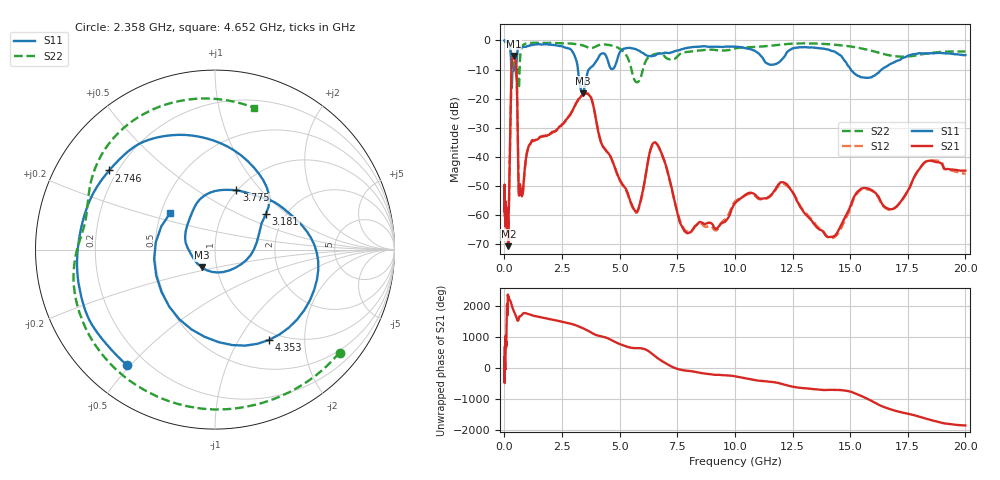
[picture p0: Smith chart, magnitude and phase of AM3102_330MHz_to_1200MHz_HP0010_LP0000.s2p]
! Date/Time: Tue, Sep 11, 2018 5:10 PM
! Network Analyzer: Agilent Technologies E8362B Rev: A.07.50.63
! Sweep from 0.010 to 20.000 GHz, 1601 Points, Sweep Type: LOG
! Power Supply: 4.949 V, 0.000 A
# Hz S DB R 50
!freq MagS11 AngS11 MagS21 AngS21 MagS12 AngS12 MagS22 AngS22
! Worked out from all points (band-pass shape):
!   1601 points, 10 MHz to 20 GHz, reference 50 ohm
!   highest |S21| = -5.33 dB at 402.8 MHz (marker M1); lowest = -70.8 dB at 172.9 MHz (marker M2)
!   |S21| within 3 dB of the highest: 318.5 MHz to 511.9 MHz (193.4 MHz wide, 46.6 % of centre)
!   lowest |S11| = -18.1 dB at 3.4 GHz (marker M3), VSWR 1.28, Z = 42.3 - j8.53 ohm
!   |S11| at or under -10 dB: 298 MHz to 356.1 MHz (58.13 MHz wide, 17.8 % of centre); 3.19 GHz to 3.661 GHz (470.9 MHz wide, 13.7 % of centre); 15.03 GHz to 16.37 GHz (1.347 GHz wide, 8.58 % of centre)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
!   |S22| runs from -16.6 to -0.2 dB; largest |S21 - S12| = 0.0066
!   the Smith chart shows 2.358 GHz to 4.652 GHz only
!   S11 on the Smith chart (normalised r, x): 2.358 GHz: 0.13, -0.49; 2.746 GHz: 0.17, +0.32; 3.181 GHz: 1.59, +0.72; 3.775 GHz: 0.99, +0.75; 4.353 GHz: 0.88, -1.36; 4.652 GHz: 0.56, +0.26
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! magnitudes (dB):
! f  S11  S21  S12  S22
! 10 MHz  0.0  -52.3  -49.6  -0.2
! 35.55 MHz  0.0  -61.4  -61.0  -0.3
! 126.4 MHz  -0.4  -63.0  -64.0  -0.7
! 172.9 MHz  -0.8  -70.8  -64.5  -1.0
! 307.3 MHz  -13.9  -10.5  -10.5  -6.9
! 402.8 MHz  -10.3  -5.3  -5.4  -7.9
! 447.2 MHz  -8.9  -5.8  -5.8  -7.4
! 530.6 MHz  -7.1  -11.5  -11.5  -12.5
! 635.6 MHz  -2.2  -53.4  -53.6  -15.9
! 1.59 GHz  -1.4  -33.1  -33.1  -0.8
! 2.358 GHz  -1.8  -29.9  -30.2  -0.9
! 2.746 GHz  -2.7  -26.7  -26.8  -1.0
! 3.181 GHz  -9.2  -20.6  -20.8  -1.3
! 3.4 GHz  -18.1  -18.6  -18.7  -1.7
! 3.775 GHz  -9.1  -20.0  -20.0  -2.6
! 4.353 GHz  -4.6  -37.4  -37.3  -1.4
! 4.652 GHz  -9.8  -40.8  -40.8  -1.7
! 5.652 GHz  -2.9  -58.5  -58.9  -13.7
! 6.549 GHz  -5.1  -35.1  -35.4  -4.6
! 7.958 GHz  -2.5  -66.4  -65.8  -3.9
! 14.07 GHz  -3.2  -67.7  -67.8  -1.3
! 20 GHz  -5.0  -44.8  -45.9  -3.8
